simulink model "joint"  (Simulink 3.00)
settings: Solver=ode45  StartTime=0.0  StopTime=5  FixedStep=.01  MaxStep=0.01  RelTol=1e-3
libraries: simulink3 x1

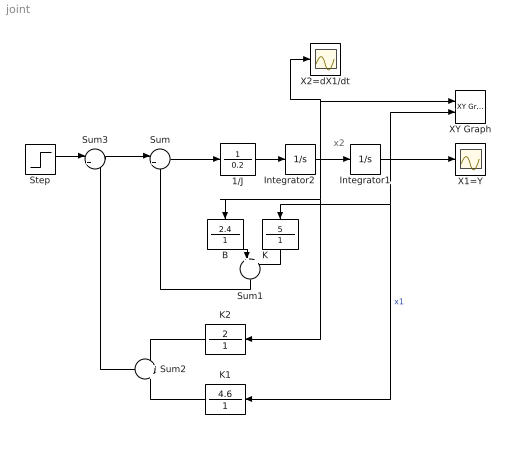
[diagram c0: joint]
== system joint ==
  note: x2
  1/J : TransferFcn  Numerator=1  Denominator=0.2
  B : TransferFcn  Orientation=down  Numerator=2.4  Denominator=1
  Integrator1 : Integrator  ExternalReset=none  InitialConditionSource=internal  InitialCondition=0  LimitOutput=off  UpperSaturationLimit=inf  LowerSaturationLimit=-inf  ShowSaturationPort=off  ShowStatePort=off  AbsoluteTolerance=auto
  Integrator2 : Integrator  ExternalReset=none  InitialConditionSource=internal  InitialCondition=0  LimitOutput=off  UpperSaturationLimit=inf  LowerSaturationLimit=-inf  ShowSaturationPort=off  ShowStatePort=off  AbsoluteTolerance=auto
  K : TransferFcn  Orientation=down  Numerator=5  Denominator=1
  K1 : TransferFcn  Orientation=left  Numerator=4.6  Denominator=1
  K2 : TransferFcn  Orientation=left  Numerator=2  Denominator=1
  Step : Step  Time=0  Before=0  After=1  SampleTime=0.001
  Sum : Sum  Inputs=|+-  SaturateOnIntegerOverflow=on
  Sum1 : Sum  Orientation=down  Inputs=+||+  SaturateOnIntegerOverflow=on
  Sum2 : Sum  Orientation=left  Inputs=+||+  SaturateOnIntegerOverflow=on
  Sum3 : Sum  Inputs=|++  SaturateOnIntegerOverflow=on
  X1=Y : Scope
  X2=dX1/dt : Scope
  XY Graph : simulink3/Sinks/XY Graph  xmin=-1  xmax=1  ymin=-1  ymax=1  st=.1
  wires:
  Sum/1 -> 1/J/1
  Sum1/1 -> Sum/2
  Integrator1/1 -> X1=Y/1, XY Graph/2, K1/1, K/1  "x1"
  1/J/1 -> Integrator2/1
  Integrator2/1 -> X2=dX1/dt/1, XY Graph/1, Integrator1/1, K2/1, B/1
  Sum2/1 -> Sum3/2
  Sum3/1 -> Sum/1
  Step/1 -> Sum3/1
  B/1 -> Sum1/1
  K/1 -> Sum1/2
  K2/1 -> Sum2/1
  K1/1 -> Sum2/2
